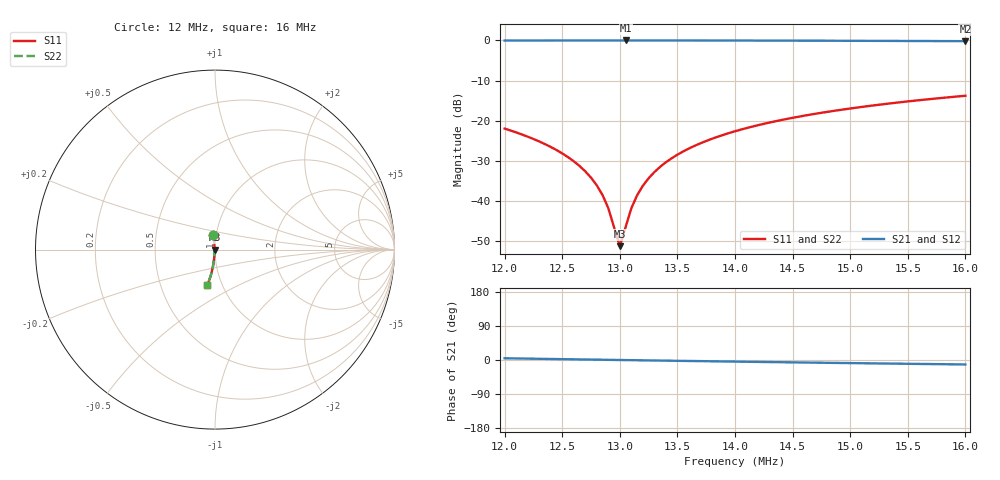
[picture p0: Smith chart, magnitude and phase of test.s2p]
# MHz S RI R 50
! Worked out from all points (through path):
!   81 points, 12 MHz to 16 MHz, reference 50 ohm
!   highest |S21| = -0.02 dB at 13.05 MHz (marker M1); lowest = -0.2 dB at 16 MHz (marker M2)
!   lowest |S11| = -51.2 dB at 13 MHz (marker M3), VSWR 1.01, Z = 49.7 - j0.00119 ohm
!   |S11| at or under -10 dB: start of sweep to end of sweep
!   |S22| runs from -51.2 to -13.8 dB; largest |S21 - S12| = 0
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12  -0.00925 0.0792  0.9907 0.0792  0.9907 0.0792  -0.00925 0.0792
12.2  -0.00688 0.0629  0.9931 0.0629  0.9931 0.0629  -0.00688 0.0629
12.4  -0.00506 0.0469  0.9949 0.0469  0.9949 0.0469  -0.00506 0.0469
12.55  -0.00405 0.035  0.9959 0.035  0.9959 0.035  -0.00405 0.035
12.7  -0.00334 0.0232  0.9967 0.0232  0.9967 0.0232  -0.00334 0.0232
12.8  -0.00302 0.0154  0.997 0.0154  0.997 0.0154  -0.00302 0.0154
12.85  -0.0029 0.0115  0.9971 0.0115  0.9971 0.0115  -0.0029 0.0115
12.9  -0.00282 0.00767  0.9972 0.00767  0.9972 0.00767  -0.00282 0.00767
13  -0.00274 -1.2e-05  0.9973 -1.2e-05  0.9973 -1.2e-05  -0.00274 -1.2e-05
13.05  -0.00275 -0.00383  0.9973 -0.00383  0.9973 -0.00383  -0.00275 -0.00383
13.1  -0.00278 -0.00763  0.9972 -0.00763  0.9972 -0.00763  -0.00278 -0.00763
13.15  -0.00285 -0.0114  0.9972 -0.0114  0.9972 -0.0114  -0.00285 -0.0114
13.25  -0.00306 -0.019  0.9969 -0.019  0.9969 -0.019  -0.00306 -0.019
13.35  -0.00338 -0.0264  0.9966 -0.0264  0.9966 -0.0264  -0.00338 -0.0264
13.45  -0.00382 -0.0338  0.9962 -0.0338  0.9962 -0.0338  -0.00382 -0.0338
13.6  -0.00466 -0.0448  0.9953 -0.0448  0.9953 -0.0448  -0.00466 -0.0448
13.8  -0.00615 -0.0593  0.9939 -0.0593  0.9939 -0.0593  -0.00615 -0.0593
14  -0.00802 -0.0734  0.992 -0.0734  0.992 -0.0734  -0.00802 -0.0734
14.3  -0.0115 -0.0941  0.9885 -0.0941  0.9885 -0.0941  -0.0115 -0.0941
14.7  -0.0173 -0.1208  0.9827 -0.1208  0.9827 -0.1208  -0.0173 -0.1208
15.35  -0.0293 -0.1617  0.9707 -0.1617  0.9707 -0.1617  -0.0293 -0.1617
16  -0.044 -0.1995  0.956 -0.1995  0.956 -0.1995  -0.044 -0.1995
